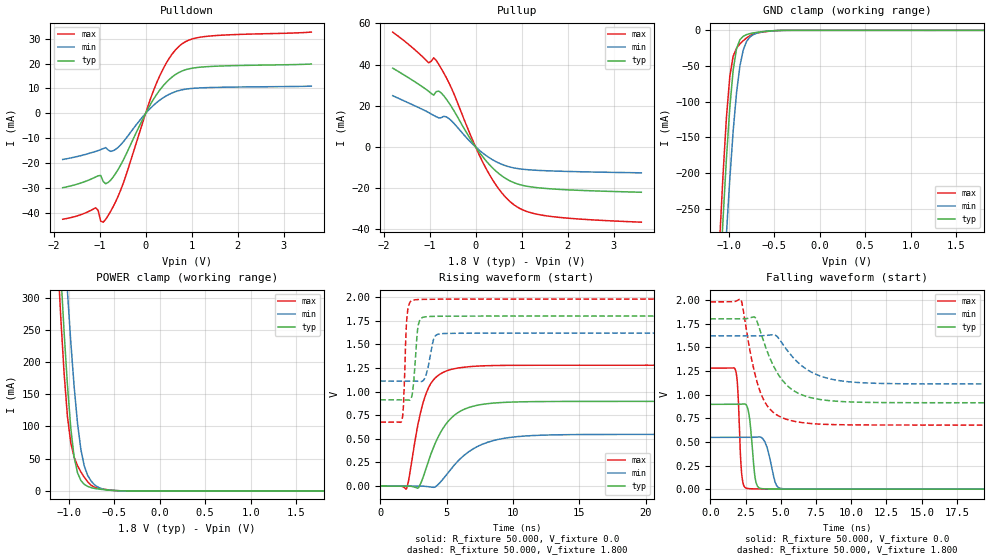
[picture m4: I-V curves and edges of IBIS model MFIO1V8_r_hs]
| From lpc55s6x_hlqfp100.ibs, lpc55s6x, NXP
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|   Model MFIO1V8_r_hs
[Model] MFIO1V8_r_hs
Model_type I/O
Polarity   Non-Inverting
Enable   Active-Low
Vinl =  0.540V
Vinh =  1.260V
Vmeas =  0.900V
Cref =  0.0F
Rref =  100.000
Vref =  0.0V
C_comp   2.019pF   1.989pF   2.068pF
C_comp_pullup   1.198pF   1.161pF   1.251pF
C_comp_pulldown   0.670pF   0.661pF   0.684pF
[Model Spec]
Vinh   1.260V   1.134V   1.386V
Vinl   0.540V   0.486V   0.594V
Vmeas   0.900V   0.810V   0.990V
Vref   0.0V   0.0V   0.0V
Cref   0.0F   0.0F   0.0F
Rref   100.000   100.000   100.000
[Temperature Range]   25.000   0.125k   -40.000
[Voltage Range]   1.800V   1.620V   1.980V
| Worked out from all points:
|   slope of the pulldown table from 0 to 0.27 V, typ, clamps not added: 32.2 ohm
|   slope of the pullup table from 0 to 0.27 V, typ, clamps not added: 34.3 ohm
|   GND clamp passes 1 mA (typ) near -0.56 V on its own axis
|   POWER clamp passes 1 mA (typ) near -0.54 V on its own axis
|   rising waveform, R_fixture 50.000, V_fixture 0.0: 20-80 % time 1.89ns typ, 2.67ns min, 1.22ns max; typ from 0 V to 0.897 V
|   rising waveform, R_fixture 50.000, V_fixture 1.800: 20-80 % time 275ps typ, 424ps min, 192ps max; typ from 0.913 V to 1.8 V
|   falling waveform, R_fixture 50.000, V_fixture 0.0: 20-80 % time 312ps typ, 502ps min, 221ps max; typ from 0.897 V to 0 V
|   falling waveform, R_fixture 50.000, V_fixture 1.800: 20-80 % time 1.84ns typ, 2.29ns min, 1.28ns max; typ from 1.8 V to 0.913 V
[Pulldown]
|Voltage   I(typ)   I(min)   I(max)
-1.8V     -29.75mA   -18.45mA   -42.39mA
-1.085V   -25.48mA   -15.2mA    -37.79mA
-1.03V    -24.99mA   -14.87mA   -38.88mA
-975mV    -24.83mA   -14.51mA   -43.15mA
-865mV    -28.18mA   -13.68mA   -42.43mA
-700mV    -25.38mA   -14.92mA   -37.23mA
-480mV    -18.54mA   -11.29mA   -27.73mA
235mV     7.474mA    4.265mA    12.03mA
510mV     13.55mA    7.648mA    22.01mA
785mV     16.96mA    9.446mA    27.8mA
1.39V     18.81mA    10.38mA    31.01mA
3.6V      19.8mA     10.93mA    32.61mA
[Pullup]
|Voltage   I(typ)   I(min)   I(max)
-1.8V     38.29mA    24.9mA     55.82mA
-1.02V    27.05mA    16.71mA    40.87mA
-910mV    25.14mA    15.31mA    43.32mA
-855mV    26.89mA    14.69mA    42.04mA
-745mV    26.24mA    14.22mA    38.06mA
-580mV    21.45mA    13.82mA    31.22mA
190mV     -5.761mA   -3.564mA   -8.914mA
520mV     -13.24mA   -7.997mA   -20.92mA
795mV     -17.02mA   -10.03mA   -27.47mA
1.07V     -18.92mA   -10.95mA   -31.04mA
1.51V     -20.18mA   -11.56mA   -33.41mA
3.6V      -22.04mA   -12.6mA    -36.6mA
[GND_clamp]
|Voltage   I(typ)   I(min)   I(max)
-1.8V     -2.463A    -2.494A    -2.446A
-1.097V   -357.7mA   -460.7mA   -294.8mA
-1.06V    -264.9mA   -370.9mA   -202.5mA
-1.023V   -180.4mA   -286.3mA   -122.9mA
-986mV    -108.7mA   -208.9mA   -65.05mA
-949mV    -56.06mA   -141.4mA   -36.24mA
-912mV    -25.87mA   -87.65mA   -25.01mA
-875mV    -13.21mA   -49.99mA   -19.06mA
-838mV    -8.315mA   -27.44mA   -14.52mA
-764mV    -4.558mA   -9.219mA   -7.395mA
-542mV    -813.9uA   -810.7uA   -1.086mA
1.8V      0A         0A         -4.189uA
[POWER_clamp]
|Voltage   I(typ)   I(min)   I(max)
-1.8V     2.577A     2.626A     2.553A
-1.123V   442.8mA    582.7mA    371.7mA
-1.086V   342mA      487.8mA    272.2mA
-1.049V   248.2mA    396.7mA    184.1mA
-1.012V   164.7mA    310.5mA    115.9mA
-975mV    97.36mA    231.1mA    74.42mA
-938mV    52.18mA    161.5mA    52.15mA
-864mV    16.11mA    64.03mA    29.39mA
-790mV    7.037mA    24.23mA    14.18mA
-679mV    3.116mA    6.059mA    4.361mA
-494mV    554.4uA    627.7uA    712.3uA
1.8V      0A         0A         4.198uA
[Ramp]
| variable   typ   min   max
dV/dt_r   0.538/1.890n   0.328/2.679n   0.768/1.212n
dV/dt_f   0.532/1.835n   0.305/2.290n   0.781/1.279n
R_load = 50.000
[Rising Waveform]
R_fixture= 50.000
V_fixture= 0.0
V_fixture_min= 0.0
V_fixture_max= 0.0
|time   V(typ)   V(min)   V(max)
0s        6.721nV    117.6nV    4.416nV
1.96ns    159.3uV    -64.23nV   -31.68mV
2.88ns    -16.7mV    137.2uV    679.8mV
3.65ns    271.3mV    -6.648mV   1.047V
4.17ns    464.1mV    -6.666mV   1.149V
4.97ns    661.3mV    117.4mV    1.218V
6.59ns    827.9mV    355.9mV    1.263V
9.2ns     885.2mV    502.7mV    1.278V
13.7ns    896.1mV    543.8mV    1.28V
100ns     896.7mV    547.4mV    1.28V
[Rising Waveform]
R_fixture= 50.000
V_fixture= 1.800
V_fixture_min= 1.620
V_fixture_max= 1.980
|time   V(typ)   V(min)   V(max)
0s        913.3mV    1.112V     677.7mV
1.62ns    913.3mV    1.112V     692.6mV
1.78ns    913.6mV    1.112V     939.1mV
2.05ns    911.1mV    1.112V     1.849V
2.41ns    974.9mV    1.112V     1.967V
2.68ns    1.419V     1.111V     1.973V
3.06ns    1.773V     1.107V     1.976V
4.06ns    1.797V     1.571V     1.979V
4.8ns     1.798V     1.615V     1.98V
100ns     1.8V       1.62V      1.98V
[Falling Waveform]
R_fixture= 50.000
V_fixture= 0.0
V_fixture_min= 0.0
V_fixture_max= 0.0
|time   V(typ)   V(min)   V(max)
0s        896.7mV    547.4mV    1.28V
1.79ns    896.7mV    547.4mV    1.259V
1.94ns    896.6mV    547.4mV    1.083V
2.25ns    898.7mV    547.4mV    128mV
2.76ns    775.2mV    547.3mV    5.302mV
3.22ns    84.03mV    550.3mV    2.398mV
3.82ns    3.468mV    513.9mV    772.7uV
4.67ns    1.151mV    47.58mV    340.7uV
5.35ns    642.8uV    3.027mV    184.5uV
100ns     14.3nV     131.2nV    8.878nV
[Falling Waveform]
R_fixture= 50.000
V_fixture= 1.800
V_fixture_min= 1.620
V_fixture_max= 1.980
|time   V(typ)   V(min)   V(max)
0s        1.8V       1.62V      1.98V
2.16ns    1.8V       1.62V      2.006V
3.18ns    1.814V     1.62V      1.212V
3.84ns    1.538V     1.623V     928.3mV
4.62ns    1.264V     1.627V     794.8mV
5.16ns    1.142V     1.529V     751.1mV
7.24ns    962.9mV    1.232V     692.1mV
9.47ns    924.9mV    1.141V     680.4mV
13.33ns   914.4mV    1.115V     677.8mV
100ns     913.3mV    1.112V     677.7mV
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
